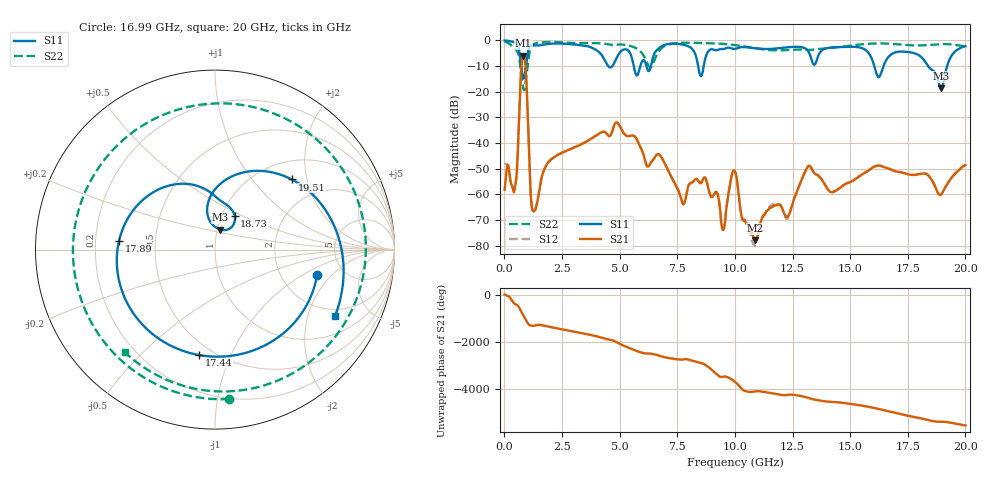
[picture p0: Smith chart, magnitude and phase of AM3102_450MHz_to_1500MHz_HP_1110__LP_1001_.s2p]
!Agilent Technologies,E8364B,MY43040894,A.07.50.67
!Agilent E8364B: A.07.50.67
!Date: Thursday, January 11, 2018 06:44:36
!Correction: S11(Full 2 Port(1,2))
!S21(Full 2 Port(1,2))
!S12(Full 2 Port(1,2))
!S22(Full 2 Port(1,2))
!S2P File: Measurements: S11, S21, S12, S22:
# Hz S  dB  R 50
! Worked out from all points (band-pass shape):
!   1601 points, 10 MHz to 20 GHz, reference 50 ohm
!   highest |S21| = -5.97 dB at 822.1 MHz (marker M1); lowest = -77.8 dB at 10.87 GHz (marker M2)
!   |S21| within 3 dB of the highest: 753.1 MHz to 904.6 MHz (151.5 MHz wide, 18.3 % of centre)
!   lowest |S11| = -18.7 dB at 18.95 GHz (marker M3), VSWR 1.26, Z = 51.7 + j11.7 ohm
!   |S11| at or under -10 dB: 5.61 GHz to 5.9 GHz (289.6 MHz wide, 5.03 % of centre); 16.05 GHz to 16.45 GHz (402.7 MHz wide, 2.48 % of centre); 18.38 GHz to 19.21 GHz (829.3 MHz wide, 4.41 % of centre)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
!   |S22| runs from -19.5 to -0.5 dB; largest |S21 - S12| = 0.0028
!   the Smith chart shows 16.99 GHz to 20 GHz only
!   S11 on the Smith chart (normalised r, x): 16.99 GHz: 3.19, -1.37; 17.44 GHz: 0.42, -0.77; 17.89 GHz: 0.30, +0.04; 18.73 GHz: 1.15, +0.46; 19.51 GHz: 1.38, +1.63; 20 GHz: 1.69, -3.00
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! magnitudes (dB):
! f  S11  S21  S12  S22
! 10 MHz  -0.1  -58.1  -47.9  -0.5
! 459.8 MHz  -0.9  -57.1  -57.0  -3.4
! 822.1 MHz  -14.9  -6.0  -6.0  -18.8
! 1.259 GHz  -2.0  -66.4  -66.3  -1.5
! 1.897 GHz  -1.5  -47.6  -47.5  -0.7
! 3.346 GHz  -2.0  -40.4  -40.4  -1.1
! 4.883 GHz  -6.7  -32.0  -32.0  -1.7
! 6.682 GHz  -3.3  -44.3  -44.3  -4.5
! 7.756 GHz  -1.7  -63.8  -63.5  -1.0
! 8.706 GHz  -7.4  -53.5  -53.6  -1.1
! 9.493 GHz  -3.5  -73.8  -73.1  -1.4
! 10.01 GHz  -3.4  -51.1  -51.0  -1.9
! 10.87 GHz  -3.1  -77.8  -80.1  -3.1
! 13.34 GHz  -8.0  -50.1  -50.2  -3.7
! 16.68 GHz  -6.4  -50.0  -50.0  -1.3
! 16.99 GHz  -4.6  -51.1  -50.9  -1.6
! 17.44 GHz  -4.5  -52.0  -51.9  -1.9
! 17.89 GHz  -5.4  -52.3  -52.3  -2.0
! 18.73 GHz  -13.2  -57.7  -57.7  -1.6
! 18.95 GHz  -18.7  -60.0  -59.8  -1.5
! 19.51 GHz  -4.7  -52.3  -52.2  -1.8
! 20 GHz  -2.3  -48.6  -48.4  -2.4
